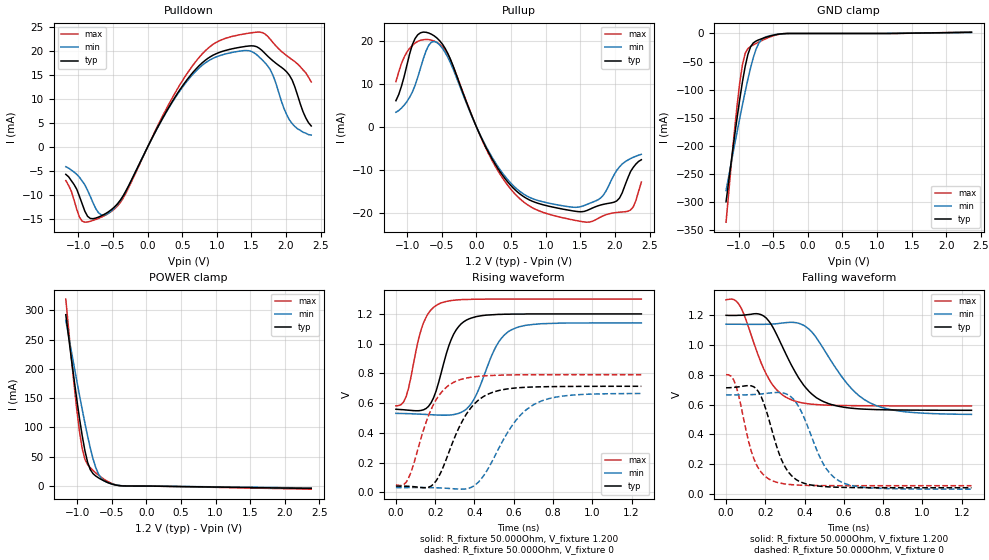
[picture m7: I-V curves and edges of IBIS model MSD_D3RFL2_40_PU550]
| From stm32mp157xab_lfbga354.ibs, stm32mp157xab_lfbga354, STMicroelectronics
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[Model] MSD_D3RFL2_40_PU550
Model_type   I/O
C_comp 2.435pF   2.348pF   2.561pF
Vinh = 820.000mV
Vinl = 380.000mV
Vmeas = 600.000mV
Vref = 600.000mV
[Model Spec]
Vinh   820.000mV   790.000mV   870.000mV
Vinl   380.000mV   350.000mV   430.000mV
Vmeas   600.000mV   570.000mV   650.000mV
Vref   600.000mV   570.000mV   650.000mV
[Temperature Range]   25.000   125.000   -40.000
[Voltage Range]   1.200V   1.140V   1.300V
[GND Clamp Reference]   0.00V   0.00V   0.00V
[Pulldown Reference]   0.00V   0.00V   0.00V
[POWER Clamp Reference]   1.200V   1.140V   1.300V
[Pullup Reference]   1.200V   1.140V   1.300V
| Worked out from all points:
|   slope of the pulldown table from 0 to 0.18 V, typ, clamps not added: 35.6 ohm
|   slope of the pullup table from 0 to 0.18 V, typ, clamps not added: 29.6 ohm
|   GND clamp passes 1 mA (typ) near -0.40 V on its own axis
|   POWER clamp passes 1 mA (typ) near -0.41 V on its own axis
|   rising waveform, R_fixture 50.000Ohm, V_fixture 1.200: 20-80 % time 91.6ps typ, 119ps min, 77.8ps max; typ from 0.559 V to 1.2 V
|   rising waveform, R_fixture 50.000Ohm, V_fixture 0: 20-80 % time 146ps typ, 180ps min, 123ps max; typ from 0.042 V to 0.713 V
|   falling waveform, R_fixture 50.000Ohm, V_fixture 1.200: 20-80 % time 165ps typ, 206ps min, 133ps max; typ from 1.2 V to 0.562 V
|   falling waveform, R_fixture 50.000Ohm, V_fixture 0: 20-80 % time 103ps typ, 128ps min, 86.3ps max; typ from 0.713 V to 0.041 V
[GND Clamp]
-1.182V   -299.3mA   -279.3mA   -335.5mA
-1.064V   -187.1mA   -201.6mA   -177.2mA
-984.9mV  -117.6mA   -151.4mA   -88.33mA
-945.5mV  -86.31mA   -127.1mA   -55.53mA
-906.1mV  -58.92mA   -103.8mA   -35.42mA
-866.7mV  -37.43mA   -81.52mA   -27.01mA
-827.3mV  -23.64mA   -60.97mA   -23.23mA
-748.5mV  -13.47mA   -27.99mA   -17.8mA
-709.1mV  -11.3mA    -17.39mA   -15.29mA
-630.3mV  -7.775mA   -7.441mA   -10.6mA
-472.7mV  -2.409mA   -2.105mA   -3.132mA
2.364V    2.067mA    1.746mA    2.431mA
[Power Clamp]
-1.164V   292.4mA    282.7mA    319.1mA
-1.085V   218.6mA    231mA      220mA
-1.006V   148.4mA    180.1mA    131mA
-966.7mV  115.9mA    155.2mA    93.22mA
-927.3mV  86.08mA    130.9mA    63.88mA
-887.9mV  60.35mA    107.4mA    45.77mA
-809.1mV  27.78mA    64.33mA    31.06mA
-730.3mV  17mA       31.16mA    22.35mA
-690.9mV  13.91mA    20.33mA    18.49mA
-572.7mV  6.632mA    6.569mA    8.741mA
-336.4mV  198.8uA    376.6uA    221.3uA
2.382V    -4.134mA   -3.29mA    -5.363mA
[Pulldown]
-1.182V   -5.7mA     -4.1mA     -7mA
-945.5mV  -11.86mA   -7.1mA     -15.47mA
-866.7mV  -14.47mA   -9.06mA    -15.65mA
-709.1mV  -14.62mA   -13.73mA   -14.9mA
-551.5mV  -13.37mA   -13.65mA   -13.71mA
-354.6mV  -10.22mA   -10.29mA   -10.7mA
590.9mV   14.46mA    14.13mA    15.78mA
945.5mV   19.18mA    18.53mA    21.44mA
1.379V    20.93mA    20.13mA    23.58mA
1.773V    18.47mA    16.13mA    22.49mA
2.009V    15.7mA     6.78mA     19.1mA
2.364V    4.4mA      2.5mA      13.6mA
[Pullup]
-1.164V   6.1mA      3.409mA    10.52mA
-887.9mV  20.5mA     9.631mA    19.46mA
-730.3mV  21.97mA    17.57mA    20.3mA
-612.1mV  21.14mA    19.85mA    19.93mA
-375.8mV  15.68mA    14.87mA    15.59mA
215.2mV   -7.105mA   -6.743mA   -7.481mA
727.3mV   -16.61mA   -16.01mA   -17.94mA
1.515V    -19.67mA   -18.45mA   -21.93mA
1.791V    -18.11mA   -16.51mA   -20.91mA
1.988V    -17.45mA   -11.09mA   -19.92mA
2.264V    -9.4mA     -7.043mA   -18.57mA
2.382V    -7.6mA     -6.348mA   -12.78mA
[Ramp]
R_load=50.000Ohm
dV/dt_r   393.258mV/119.500ps  372.822mV/150.500ps  433.617mV/100.500ps
dV/dt_f   393.258mV/135.000ps  372.732mV/169.000ps  433.617mV/110.000ps
[Rising waveform]
R_fixture=50.000Ohm
V_fixture=1.200
V_fixture_min=1.140
V_fixture_max=1.300
0s        559mV      531.2mV    581.9mV
52ps      554mV      529.8mV    644.4mV
154ps     564.3mV    523.9mV    1.179V
230ps     800.9mV    519.2mV    1.274V
281ps     1.026V     520.9mV    1.29V
332ps     1.133V     537.7mV    1.296V
396ps     1.177V     622.2mV    1.299V
524ps     1.197V     1.013V     1.3V
588ps     1.199V     1.093V     1.3V
1.25ns    1.2V       1.14V      1.3V
[Rising waveform]
R_fixture=50.000Ohm
V_fixture=0
0s        42.02mV    31.93mV    50.03mV
64ps      40.74mV    32.3mV     95.29mV
192ps     56.6mV     31.47mV    592.7mV
307ps     394.4mV    22.92mV    748mV
371ps     549.5mV    27.44mV    771.9mV
447ps     645.4mV    112.3mV    783.2mV
600ps     700.8mV    464.8mV    790.1mV
703ps     708.8mV    591.5mV    791.3mV
894ps     712.4mV    653.7mV    791.7mV
1.25ns    713.4mV    664.9mV    791.7mV
[Falling waveform]
R_fixture=50.000Ohm
V_fixture=1.200
V_fixture_min=1.140
V_fixture_max=1.300
0s        1.2V       1.14V      1.304V
77ps      1.2V       1.14V      1.249V
192ps     1.195V     1.139V     839.5mV
256ps     1.075V     1.143V     701.8mV
320ps     898.6mV    1.152V     639.4mV
396ps     728.9mV    1.132V     609.6mV
460ps     646.2mV    1.049V     600.2mV
613ps     579.9mV    746.7mV    593.4mV
741ps     567.4mV    606.7mV    592.1mV
1.25ns    561.7mV    534.1mV    591.1mV
[Falling waveform]
R_fixture=50.000Ohm
V_fixture=0
0s        712.9mV    665.5mV    801mV
52ps      717.2mV    665.2mV    721.3mV
115ps     727.7mV    666mV      351.2mV
154ps     706.2mV    668.7mV    198.6mV
230ps     445mV      678.8mV    91.78mV
281ps     234mV      680.5mV    71.11mV
345ps     108.4mV    634.3mV    61.03mV
498ps     49.39mV    195.4mV    55.73mV
588ps     44.07mV    79.29mV    55.39mV
1.25ns    41.34mV    31.85mV    55.21mV
